TEXTLIST TextList_Recipe
  100 = ' 配方保存路径:' | chinese: ' 配方保存路径:' | english: ' Recipe Save Path:'
  101 = ' 当前配方名:' | chinese: ' 当前配方名:' | english: ' Current Recipe:'
  102 = ' 另存配方名:' | chinese: ' 另存配方名:' | english: ' Save as Recipe:'
  103 = ' 上载配方名:' | chinese: ' 上载配方名:' | english: ' Upload Recipe:'
  110 = '刷新' | chinese: '刷新' | english: 'FlashList'
  111 = '上载并激活' | chinese: '上载并激活' | english: 'LoadRecipe'
  112 = '保存' | chinese: '保存' | english: 'SaveRecipe'
  113 = '另存为...' | chinese: '另存为...' | english: 'SaveRecipeAs'
  114 = '删除' | chinese: '删除' | english: 'DeleteRecipe'
  119 = '从USB导入' | chinese: '从USB导入' | english: 'LoadFromUSB'
  120 = '确定' | chinese: '确定' | english: 'OK'
  121 = '取消' | chinese: '取消' | english: 'Cancel'
  118 = '导出到USB' | chinese: '导出到USB' | english: 'SaveToUSB'
   = ''
END_TEXTLIST
